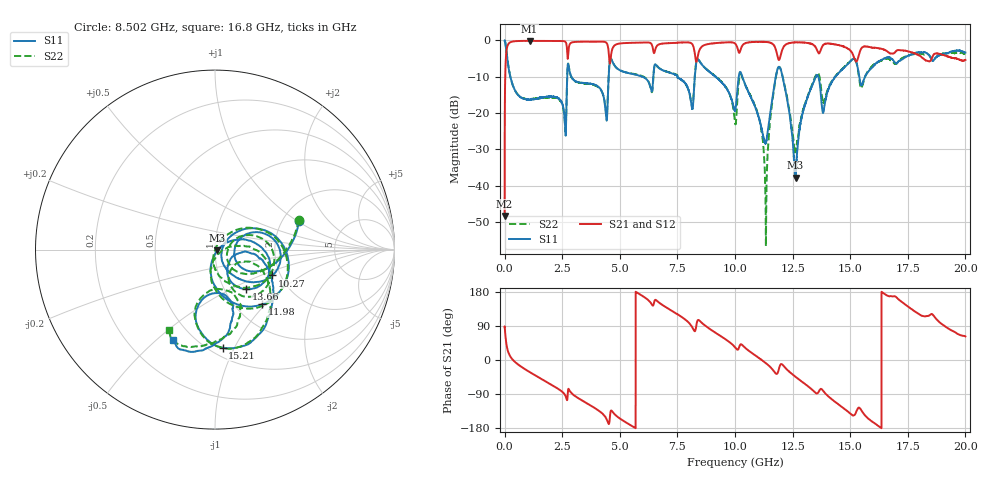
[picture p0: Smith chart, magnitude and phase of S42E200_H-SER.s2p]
!{S42E200}
!Johanson Technology Inc.
!www.johansontechnology.com
!Test Board Conditions:
!Substrate Type  RO4350B
!Substrate Thickness  50 mil
!Substrate Dk  3.66
!TL Type: GCPW
!TL Trace Width  60 mil
!TL Gap  10 mil
!Electrode orientation  Horizontal
!DUT TOPOLOGY	SERIES
!Mounting Pad LxW  14x55 mil
! Created Wed Nov 25 22:04:14 2020
# khz S ma R 50
! 2 Port Network Data from SP1.SP block
! freq  magS11  angS11  magS21  angS21  magS12  angS12  magS22  angS22
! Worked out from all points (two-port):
!   20001 points, 300 kHz to 20 GHz, reference 50 ohm
!   highest |S21| = -0.12 dB at 1.082 GHz (marker M1); lowest = -48.3 dB at 300 kHz (marker M2)
!   |S21| within 3 dB of the highest: 77.29 MHz to 2.716 GHz (2.638 GHz wide, 189 % of centre); 4.644 GHz to 6.463 GHz (1.818 GHz wide, 32.7 % of centre)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
!   lowest |S11| = -37.8 dB at 12.63 GHz (marker M3), VSWR 1.03, Z = 51.2 - j0.485 ohm
!   |S11| at or under -10 dB: 248.4 MHz to 2.717 GHz (2.468 GHz wide, 166 % of centre); 2.896 GHz to 4.517 GHz (1.621 GHz wide, 43.7 % of centre); 10.32 GHz to 11.77 GHz (1.449 GHz wide, 13.1 % of centre)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
!   |S22| runs from -56.7 to 0.0 dB; largest |S21 - S12| = 0.017
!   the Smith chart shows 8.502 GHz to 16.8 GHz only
!   S11 on the Smith chart (normalised r, x): 8.502 GHz: 2.45, +1.03; 10.27 GHz: 1.82, -0.60; 11.98 GHz: 1.32, -0.96; 13.66 GHz: 1.26, -0.60; 15.21 GHz: 0.58, -0.90; 16.8 GHz: 0.39, -0.57
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300  0.9956 -0.4  0.003829 88.4  0.003779 90.0  0.9972 -0.5
148300  0.4727 -67.2  0.8775 22.8  0.8785 22.7  0.476 -67.0
1082300  0.1529 -123.1  0.9866 -31.7  0.985 -31.6  0.1554 -121.4
3334300  0.2615 160.4  0.961 -105.8  0.9604 -105.8  0.2578 168.0
4385300  0.1075 137.4  0.9449 -151.2  0.9457 -151.2  0.112 147.1
4638300  0.548 152.5  0.6823 -133.5  0.6817 -133.6  0.5515 155.2
6667300  0.426 69.8  0.8723 153.2  0.8703 153.2  0.4271 64.7
8114300  0.1273 30.0  0.9093 89.5  0.9091 89.6  0.1304 33.4
8502300  0.4938 18.8  0.7831 101.4  0.7811 101.4  0.4941 19.6
1.00003e7  0.1081 -3.7  0.9094 33.6  0.9087 33.8  0.07489 -28.2
1.02723e7  0.3511 -24.2  0.7911 41.4  0.7932 41.4  0.3322 -29.8
1.10253e7  0.0882 -59.4  0.9575 5.9  0.9589 5.9  0.08878 -94.1
1.13343e7  0.03823 -4.3  0.9539 -8.0  0.9534 -8.0  0.003685 -83.5
1.16833e7  0.2142 33.1  0.8634 -29.2  0.8637 -29.2  0.2013 36.7
1.19793e7  0.4024 -49.1  0.6194 -11.5  0.6222 -11.5  0.4064 -51.5
1.26313e7  0.01288 -21.5  0.9423 -44.5  0.9406 -44.9  0.03085 -42.6
1.33343e7  0.2321 8.0  0.8919 -77.9  0.892 -77.6  0.2413 -2.0
1.36603e7  0.2796 -52.0  0.6675 -80.7  0.6679 -80.6  0.324 -54.5
1.52123e7  0.548 -85.6  0.5371 -143.3  0.5353 -143.9  0.5404 -87.9
1.66673e7  0.5866 -107.4  0.6853 168.6  0.6709 168.6  0.5623 -113.8
1.68013e7  0.5576 -114.9  0.662 168.2  0.6477 168.7  0.5142 -120.0
2e7  0.6808 151.0  0.5389 62.2  0.5393 63.2  0.6615 149.9
